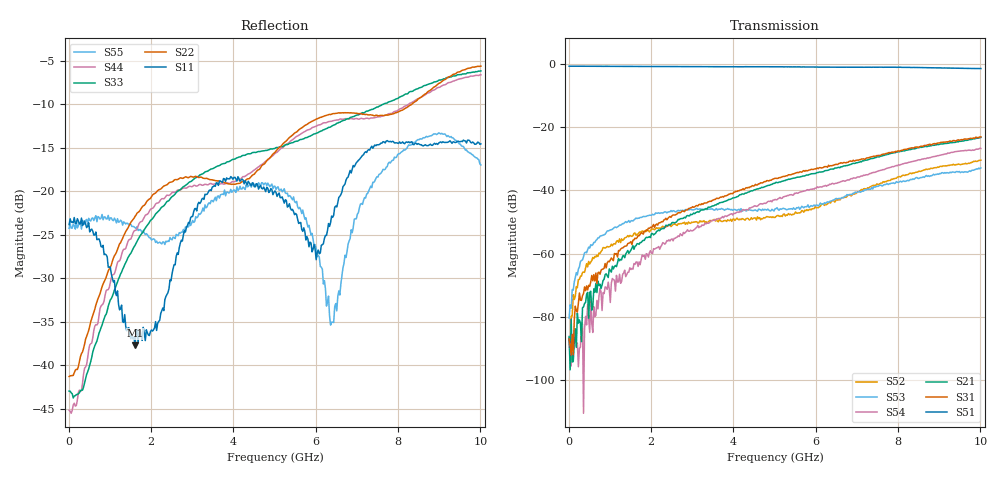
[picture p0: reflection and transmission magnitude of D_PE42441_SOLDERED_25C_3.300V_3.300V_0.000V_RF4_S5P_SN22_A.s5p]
! Device ID: PE42441
! Serial: 22
! Insertion: A
! Temp: 25C
! VDD: 3.300
! Control_Hi: 100.000
! Control_Lo: 0.000
! Logic State: RF4
! Port 1: RFC
! Port 2: RF1
! Port 3: RF2
! Port 4: RF3
! Port 5: RF4
! V1 = 3.30
! V2 = 3.30
! V3 = 0.00
! V4 = 0.00
! IDD: 1.047294e-04
! 1 Hz data is simulated
#  Hz  S  RI  R  50
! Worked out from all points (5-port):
!   401 points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, 10 MHz to 10.01 GHz, reference 50 ohm
!   strongest paths, dB at 10 MHz, 2.51 GHz, 5.01 GHz, 7.51 GHz, 10.01 GHz:
!     S51: -0.7, -0.8, -0.9, -1.0, -1.4
!     S31: -87.1, -48.0, -36.2, -29.0, -23.1
!     S21: -86.3, -50.2, -37.7, -29.4, -23.2
!     S54: -87.1, -55.4, -42.9, -33.9, -26.7
!     S53: -80.4, -46.7, -45.9, -38.7, -32.9
!     S52: -86.7, -51.2, -48.6, -38.2, -30.4
!   lowest |S11| = -37.7 dB at 1.61 GHz (marker M1), VSWR 1.03, Z = 49.6 - j1.24 ohm
!   |S11| at or under -10 dB: start of sweep to end of sweep
